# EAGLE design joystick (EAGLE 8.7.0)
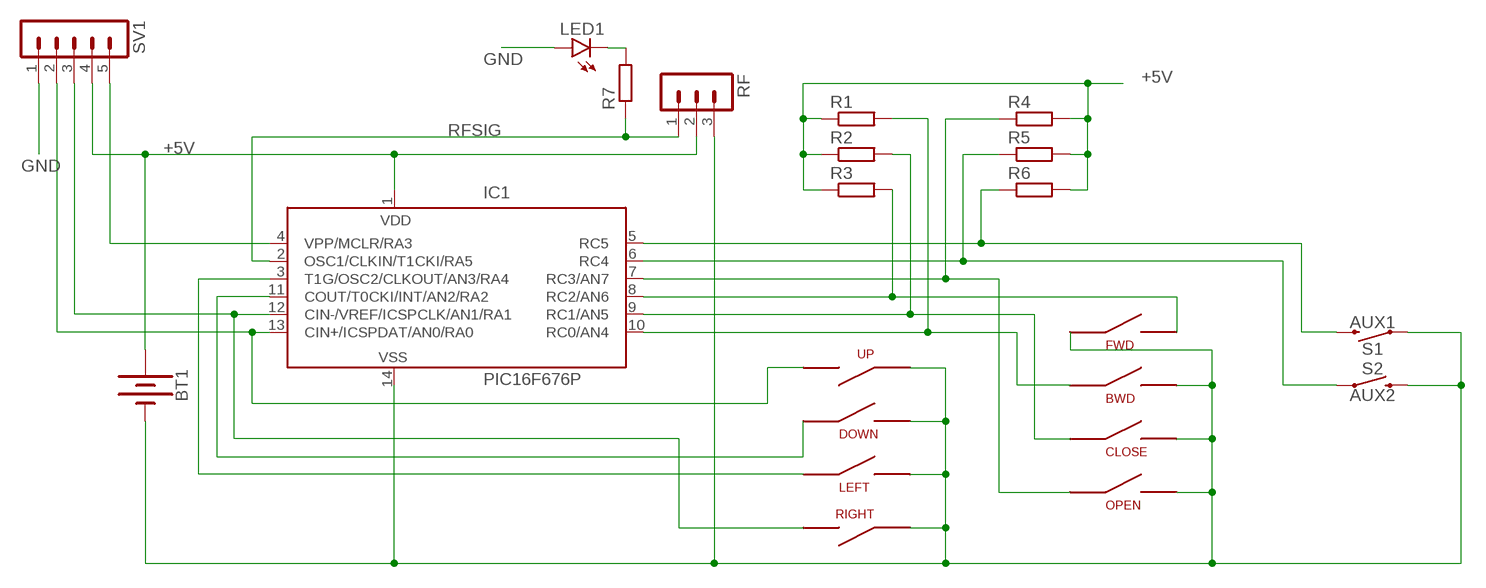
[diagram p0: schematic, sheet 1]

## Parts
BT1  BATTERY-20MM_PTH  [BATTCOM_20MM_PTH]
BWD  SWITCHMOM90  [SWITCHMOM90]
CLOSE  SWITCHMOM90  [SWITCHMOM90]
DOWN  SWITCHMOM90  [SWITCHMOM90]
FWD  SWITCHMOM90  [SWITCHMOM90]
IC1  PIC16F676P  [DIL14]
LED1  LED3MM  [LED3MM]
LEFT  SWITCHMOM90  [SWITCHMOM90]
OPEN  SWITCHMOM90  [SWITCHMOM90]
R1  R-EU_0207/10  [0207/10]
R2  R-EU_0207/10  [0207/10]
R3  R-EU_0207/10  [0207/10]
R4  R-EU_0207/10  [0207/10]
R5  R-EU_0207/10  [0207/10]
R6  R-EU_0207/10  [0207/10]
R7  R-EU_0207/10  [0207/10]
RF  MA03-1  [MA03-1]
RIGHT  SWITCHMOM90  [SWITCHMOM90]
S1  AUX1  MOMENTARY-SWITCH-SPST-PTH-6.0MM  [TACTILE_SWITCH_PTH_6.0MM]
S2  AUX2  MOMENTARY-SWITCH-SPST-PTH-6.0MM  [TACTILE_SWITCH_PTH_6.0MM]
SV1  MA05-1  [MA05-1]
UP  UP  SWITCHMOM90  [SWITCHMOM90]

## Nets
+5V: BT1.1(+) IC1.1(VDD) R1.1 R2.1 R3.1 R4.2 R5.2 R6.2 RF.2 SV1.4
GND: BT1.2(-) BWD.P$3 CLOSE.P$3 DOWN.P$3 FWD.P$1 IC1.14(VSS) LED1.A LEFT.P$3 OPEN.P$3 RF.3 RIGHT.P$1 S1.1 S2.3 SV1.1 UP.P$1
N$1: LED1.K(C) R7.2
N$2: IC1.7(RC3/AN7) OPEN.P$1 R4.1
N$3: IC1.5(RC5) R6.1 S1.3
N$4: IC1.6(RC4) R5.1 S2.1
N$6: FWD.P$3 IC1.8(RC2/AN6) R3.2
N$7: CLOSE.P$1 IC1.9(RC1/AN5) R2.2
N$9: IC1.13(CIN+/ICSPDAT/AN0/RA0) SV1.2 UP.P$3
N$10: IC1.12(CIN-/VREF/ICSPCLK/AN1/RA1) RIGHT.P$3 SV1.3
N$11: DOWN.P$1 IC1.11(COUT/T0CKI/INT/AN2/RA2)
N$12: IC1.3(T1G/OSC2/CLKOUT/AN3/RA4) LEFT.P$1
N$13: BWD.P$1 IC1.10(RC0/AN4) R1.2
N$14: IC1.4(VPP/MCLR/RA3) SV1.5
RFSIG: IC1.2(OSC1/CLKIN/T1CKI/RA5) R7.1 RF.1

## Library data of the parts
BT1 = SparkFun-Batteries:BATTERY: Battery - Single Cell; PROD_ID: BATT-09031; SF_SKU: PRT-00783
BWD CLOSE DOWN FWD LEFT OPEN RIGHT UP = MyPersonalLib:SWITCHMOM90: Momentary Switch Right Angled
IC1 = microchip:PIC16F676: 14-Pin, Flash-Based 8-Bit CMOS Microcontroller High Performance RISC CPU: * Only 35 instructions to learn - All single-cycle instructions except branches * Operating speed: - DC - 20 MHz oscillator/clock input - DC - 200 ns instruction cycle * Internal and external oscillator options - Precision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; MF: MICROCHIP; MPN: PIC16F676-I/P; OC_FARNELL: 9760512; OC_NEWARK: 54K2829
LED1 = led:LED: LED
R1-R7 = rcl:R-EU_: RESISTOR, European symbol; SPICEPREFIX: R
RF = con-lstb:MA03-1: PIN HEADER; OC_FARNELL: unknown; OC_NEWARK: unknown
S1 S2 = SparkFun-Switches:MOMENTARY-SWITCH-SPST: Momentary Switch (Pushbutton) - SPST; PROD_ID: SWCH-08441; SF_SKU: COM-00097
SV1 = con-lstb:MA05-1: PIN HEADER; OC_FARNELL: unknown; OC_NEWARK: unknown

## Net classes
0 default: width 0.4 mm, drill 0.65 mm, clearance 0.3 mm
1 GND: width 0.4 mm, drill 0.65 mm, clearance 0.3 mm

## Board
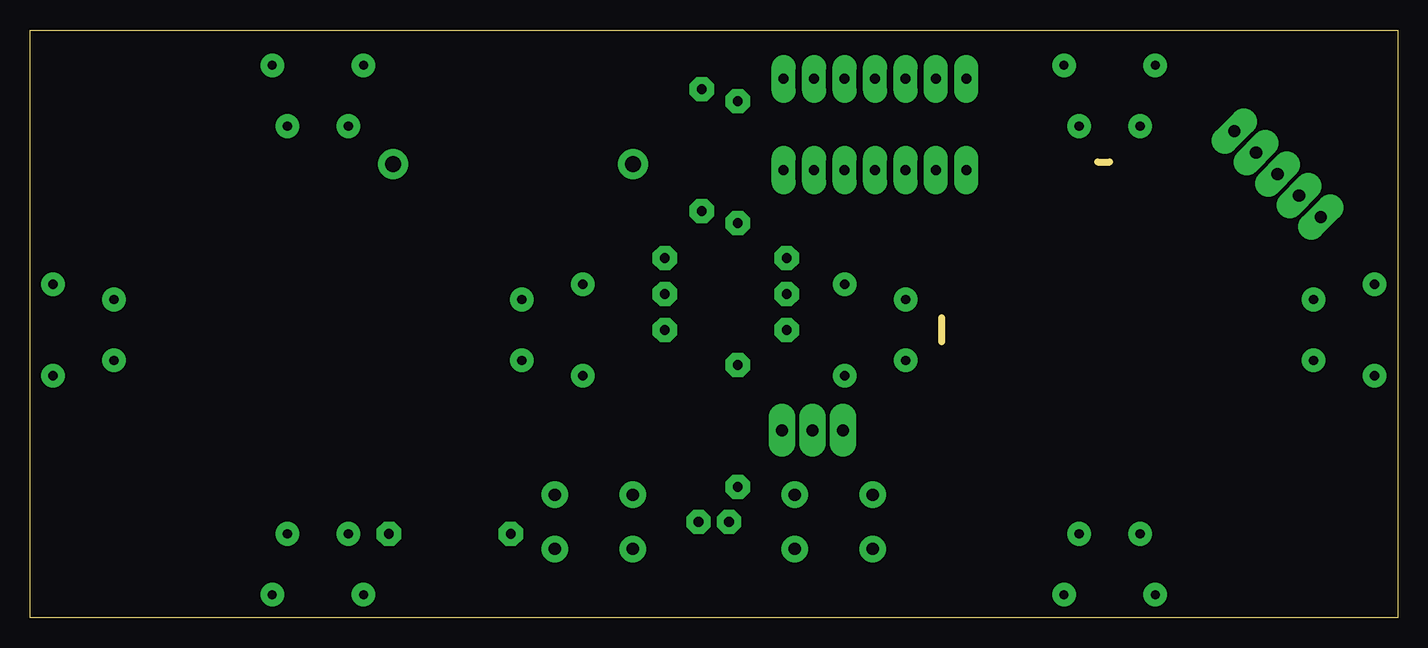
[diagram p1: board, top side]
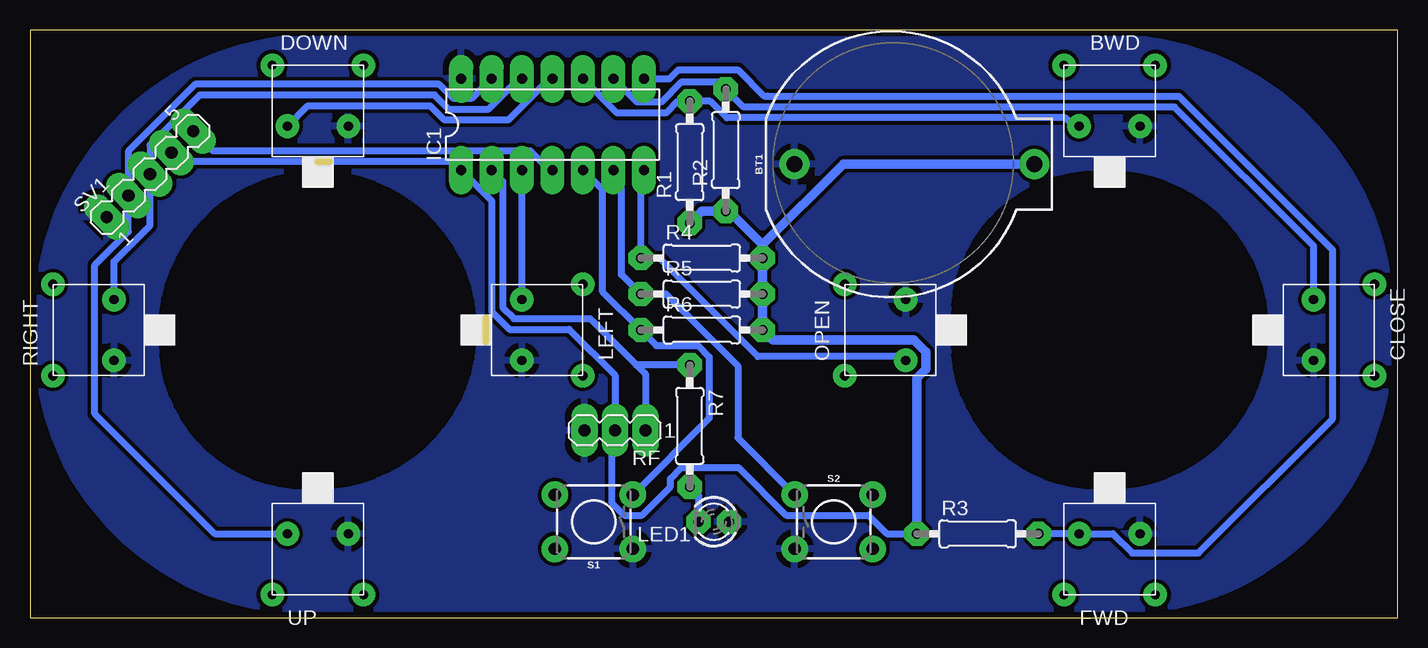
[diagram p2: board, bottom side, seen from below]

Size 114 x 49.02 mm. Coordinates in mm from the lower left corner, seen from the top.
Outline: 114,0 0,0 0,49.02 114,49.02 114,0
Copper layers (1*16): Top 0.035mm / dielectric 1.5mm / Bottom 0.035mm
Design rules "pcb_aneta8_2": minimum track width 0.5mm, minimum drill 0.6mm, track to track 0.3mm, track to pad 0.3mm, pad to pad 0.3mm, via to via 0.3mm, smd to smd 6mil, copper to edge 20mil, drill to drill 0.5mm, minimum pad ring 0.6mm, minimum via ring 0.6mm, stop-mask expansion 4mil, vias tented up to drill 0mil, thermal gap 20mil
bKeepout: 2 lines
bRestrict: area 11,24 to 11.2,25; area 77,11 to 103,37; area 11,11 to 37,37; area 0,0 to 24,23; area 90,0 to 114,23; area 90,25 to 114,49; area 0,25 to 25,49
Milling: 2 lines

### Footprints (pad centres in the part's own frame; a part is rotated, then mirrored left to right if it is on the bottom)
BATTCOM_20MM_PTH = drill 1.3: 1 11.85,0; 2 -8.15,0
SWITCHMOM90 = drill 0.762 pad 1.778: P$1 2.54,0; P$2 3.81,-5.08; P$3 -2.54,0; P$4 -3.81,-5.08
DIL14 = drill 0.813 long: 1 -7.62,-3.81; 2 -5.08,-3.81; 3 -2.54,-3.81; 4 0,-3.81; 5 2.54,-3.81; 6 5.08,-3.81; 7 7.62,-3.81; 8 7.62,3.81; 9 5.08,3.81; 10 2.54,3.81; 11 0,3.81; 12 -2.54,3.81; 13 -5.08,3.81; 14 -7.62,3.81
LED3MM = drill 0.813 octagon: A -1.27,0; K 1.27,0
0207/10 = drill 0.813 octagon: 1 -5.08,0; 2 5.08,0
MA03-1 = drill 1.016 long: 1 -2.54,0; 2 0,0; 3 2.54,0
TACTILE_SWITCH_PTH_6.0MM = drill 1.016 pad 1.88: 1 -3.251,2.261; 2 3.251,2.261; 3 -3.251,-2.261; 4 3.251,-2.261
MA05-1 = drill 1.016 long: 1 -5.08,0; 2 -2.54,0; 3 0,0; 4 2.54,0; 5 5.08,0

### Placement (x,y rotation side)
BT1  42.12,37.83 0 bottom
BWD  24,41 180 bottom
CLOSE  7,24 90 bottom
DOWN  90,41 180 bottom
FWD  24,7 0 bottom
IC1  70.44,41.14 0 bottom
LED1  57,8 180 bottom
LEFT  73,24 90 bottom
OPEN  41,24 270 bottom
R1  59,38 90 bottom
R2  56,39 90 bottom
R3  35,7 0 bottom
R4  58,30 0 bottom
R5  58,27 0 bottom
R6  58,24 0 bottom
R7  59,16 270 bottom
RF  65.24,15.63 180 bottom
RIGHT  107,24 270 bottom
S1  67,8 180 bottom
S2  47,8 0 bottom
SV1  104,37 45 bottom
UP  90,7 0 bottom

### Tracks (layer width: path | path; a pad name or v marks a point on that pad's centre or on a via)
+5V
  Bottom 0.6: R3.1 42.58,7 44.12,8.54 50.96,8.54 54.96,12.54 59.67,12.54 60.62,11.59 60.62,10.93 63,8.54 64.46,8.54 65.47,9.55 65.47,15.4 RF.2 65.24,20.24 69.05,24.05 74.03,24.05 75.49,25.51 75.49,34.76 IC1.1 78.78,38.05 101.45,38.05 SV1.4 | 52.92,30.84 R4.2
  Bottom 0.8: BT1.1 46.2,37.83 52.92,31.11 | 52.92,31.11 R4.2 R5.2 R6.2 52.07,23.15 40.3,23.15 39.31,22.16 39.31,20.76 40.08,19.99 R3.1 | 52.92,31.11 55.73,33.92 R2.1 58,33.92 R1.1
GND
  pour Bottom: 114,0 114,49 0,49 0,0
N$1
  Bottom 0.6: R7.2 58.27,10.19 LED1.K
N$2
  Bottom 0.6: IC1.7 62.82,37 63.08,36.74 R4.1 61.54,30 53.32,21.78 41.32,21.78 OPEN.P$1
N$3
  Bottom 0.6: IC1.5 66.26,35.69 66.26,27.18 R6.1 61.78,22.7 58.33,22.7 57.38,21.75 57.38,16.63 S1.3
N$4
  Bottom 0.6: IC1.6 64.7,36.67 64.7,28.62 R5.1 61,27 55,21 55,15.01 S2.1
N$6
  Bottom 0.6: R3.2 FWD.P$3 23.71,7 22.12,5.41 16.59,5.41 5.41,16.59 5.41,30.68 18.22,43.49 52.49,43.49 52.5,43.5 52.8,43.5 55,45.7 59.94,45.7 60.69,44.95 IC1.8
N$7
  Bottom 0.6: CLOSE.P$1 7,31 18.59,42.59 54.51,42.59 R2.2 56.62,44.7 59.67,44.7 61.37,43 63.41,43 IC1.9
N$9
  Bottom 0.6: UP.P$3 98.59,7 108.59,17 108.59,29.41 105.8,32.2 SV1.2 105.8,38.91 100.21,44.49 | IC1.13 77.14,43.33 78.73,43.33 79.89,44.49 100.21,44.49 | 100.21,44.49
N$10
  Bottom 0.6: RIGHT.P$3 107,29.73 104,32.73 SV1.3 104,39.43 99.84,43.59 80.26,43.59 79.1,42.43 75.75,42.43 73.23,44.95 IC1.12
N$11
  Bottom 0.6: DOWN.P$1 90.85,42.69 80.63,42.69 79.47,41.53 74.11,41.53 70.69,44.95 IC1.11
N$12
  Bottom 0.6: LEFT.P$1 72.98,26.56 IC1.3
N$13
  Bottom 0.6: BWD.P$1 27,41 27.69,41.69 55.9,41.69 57.29,43.08 R1.2 60.01,43.08 60.99,42.1 65.05,42.1 IC1.10
N$14
  Bottom 0.6: IC1.4 70.69,37.33 72.31,38.95 98.76,38.95 SV1.5
RFSIG
  Bottom 0.6: IC1.2 74.59,36.4 74.59,25.88 73.66,24.95 67.31,24.95 63.44,21.08 | RF.1 62.7,20.34 63.44,21.08 | R7.1 63.44,21.08

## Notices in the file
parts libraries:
SparkFun-Batteries: Licensing: Creative Commons ShareAlike 4.0 International - https://creativecommons.org/licenses/by-sa/4.0
